DATA_BLOCK DB 62
VERSION : 0.1


  STRUCT
   Messwert : REAL  := 1.500000e+002;
   Messwert1 : REAL  := 1.200000e+002;
   Messwert2 : REAL  := 2.220000e+002;
   Messwert3 : REAL  := 1.300000e+000;
   Messwert4 : REAL  := 5.600000e+001;
   Messwert5 : REAL  := 7.800000e+001;
   Messwert6 : REAL  := 4.670000e+002;
   Messwert7 : REAL  := 1.200000e+001;
   Messwert8 : REAL  := 1.330000e+002;
   Messwert9 : REAL  := 1.458000e+003;
   Messwert10 : REAL  := 1.200000e+001;
   Messwert11 : REAL  := 1.500000e+000;
   Messwert12 : REAL  := 4.560000e+002;
   Messwert13 : REAL  := 1.235000e+003;
   Messwert14 : REAL  := 5.000000e-001;
   Messwert15 : REAL  := 1.250000e+001;
   Messwert16 : REAL  := 1.355000e+002;
   Messwert17 : REAL  := 2.225000e+002;
   Messwert18 : REAL  := 1.236800e+003;
   Messwert19 : REAL  := 1.270000e+001;
   Messwert20 : REAL  := 5.600000e+001;
   Messwert21 : REAL  := 6.600000e-001;
   Messwert22 : REAL  := 4.500000e+001;
   Messwert23 : REAL  := 4.560000e+002;
   Messwert24 : REAL  := 1.235000e+003;
   Messwert25 : REAL  := 1.236000e+003;
   Messwert26 : REAL  := 1.120000e+002;
   Messwert27 : REAL  := 2.350000e+002;
   Messwert28 : REAL  := 2.350000e+001;
   Messwert29 : REAL  := 5.000000e-001;
  END_STRUCT ;
BEGIN
   Messwert := 1.500000e+002;
   Messwert1 := 1.200000e+002;
   Messwert2 := 2.220000e+002;
   Messwert3 := 1.300000e+000;
   Messwert4 := 5.600000e+001;
   Messwert5 := 7.800000e+001;
   Messwert6 := 4.670000e+002;
   Messwert7 := 1.200000e+001;
   Messwert8 := 1.330000e+002;
   Messwert9 := 1.458000e+003;
   Messwert10 := 1.200000e+001;
   Messwert11 := 1.500000e+000;
   Messwert12 := 4.560000e+002;
   Messwert13 := 1.235000e+003;
   Messwert14 := 5.000000e-001;
   Messwert15 := 1.250000e+001;
   Messwert16 := 1.355000e+002;
   Messwert17 := 2.225000e+002;
   Messwert18 := 1.236800e+003;
   Messwert19 := 1.270000e+001;
   Messwert20 := 5.600000e+001;
   Messwert21 := 6.600000e-001;
   Messwert22 := 4.500000e+001;
   Messwert23 := 4.560000e+002;
   Messwert24 := 1.235000e+003;
   Messwert25 := 1.236000e+003;
   Messwert26 := 1.120000e+002;
   Messwert27 := 2.350000e+002;
   Messwert28 := 2.350000e+001;
   Messwert29 := 5.000000e-001;
END_DATA_BLOCK

